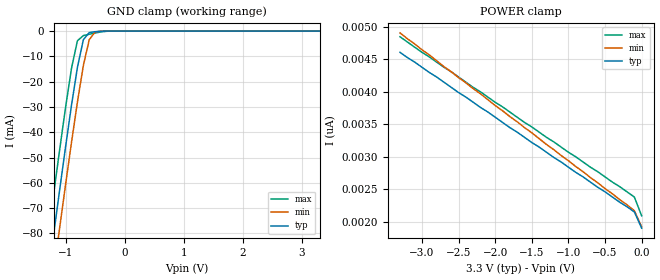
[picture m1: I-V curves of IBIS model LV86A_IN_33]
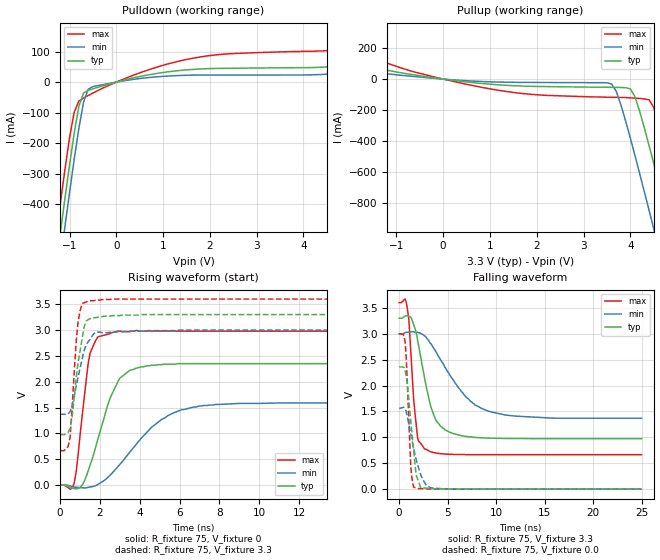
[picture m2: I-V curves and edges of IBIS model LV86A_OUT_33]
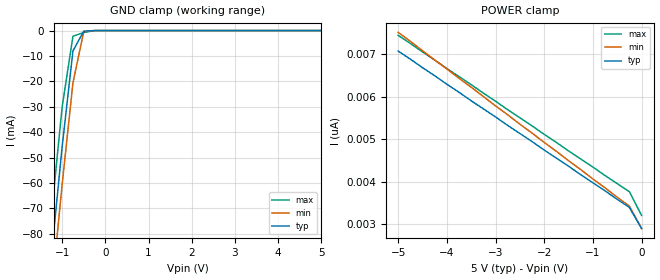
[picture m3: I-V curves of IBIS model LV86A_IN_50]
| TEXAS INSTRUMENTS INCORPORATED
| Standard Linear and Logic Group
| IBIS Model of SN74LV86A
| QUADRUPLE 2-INPUT EXCLUSIVE-OR GATE
| SOIC 14-pin (D), SOP 14-pin (NS), SSOP 14-pin (DB), TSSOP 14-pin (PW)
| and TVSOP 14-pin (DGV) Package
[IBIS Ver]   3.2
[Comment Char]  |_char
[File Name]   lv86a.ibs
[File Rev]   2.0 H_die
[Date]   May 24, 2000
[Source]   Data created from HSPICE simulations at TI-SLL.
[Notes]   The following is an IBIS list for the LV86A.
|   Please contact sllibis@ti.com with questions and
|   comments concerning SLL IBIS models.
[Disclaimer] Property of Texas Instruments Incorporated.  Unauthorized
   reproduction and/or distribution is strictly prohibited.
   This product is protected under copyright law.
   Created 2000, (C) Copyright 2000, Texas Instruments Inc.,
   All Rights Reserved.
   UNLESS THERE IS A SIGNED, WRITTEN AGREEMENT TO THE
   CONTRARY, TEXAS INSTRUMENTS () IS PROVIDING THE IBIS
   MODELS  AND WITHOUT ANY WARRANTY, EXPRESSED OR
   IMPLIED.  TI assumes no liability for:
   1) the accuracy of the IBIS models provided to your
   company;
   2) the proper functioning of these IBIS Models in your
   design or for any resulting applications; or
   3) infringement of patents, copyrights or intellectual
   property rights resulting from your use of these IBIS
   models.
   TI provides IBIS Models as a service to our customers.
   You and your company shall not distribute, sell or give
   these models to anyone else without prior written
   permission from TI.
   TI reserves the right to make changes to our products or
   to discontinue any semiconductor product or service
   without notice, and advises our customers to obtain the
   latest version of relevant information to verify, before
   placing orders, that the information being relied on is
   current.
   Please be aware that your receipt and use of the IBIS
   information provided shall serve as acceptance of these
   terms and conditions.  If you do not accept these terms,
   you should return or destroy the IBIS models and any
   other accompanying information immediately.
|   Component LV86A_D
[Component]   LV86A_D
[Manufacturer]  Texas Instruments, Inc.
[Package]
|   typ   min   max
R_pkg   0.031   0.028   0.034
L_pkg   3.109nH   2.462nH   3.889nH
C_pkg   0.473pF   0.363pF   0.628pF
[Pin]   signal_name   model_name   R_pin   L_pin   C_pin
1   1A   LV86A_IN   0.033   3.854nH   0.622pF
2   1B   LV86A_IN   0.032   3.188nH   0.473pF
3   1Y   LV86A_OUT   0.028   2.462nH   0.377pF
4   2A   LV86A_IN   0.031   2.596nH   0.363pF
5   2B   LV86A_IN   0.028   2.521nH   0.372pF
6   2Y   LV86A_OUT   0.034   3.250nH   0.476pF
7   GND   GND   0.034   3.889nH   0.628pF
8   3Y   LV86A_OUT   0.034   3.889nH   0.628pF
9   3A   LV86A_IN   0.034   3.250nH   0.476pF
10   3B   LV86A_IN   0.028   2.521nH   0.372pF
11   4Y   LV86A_OUT   0.031   2.596nH   0.364pF
12   4A   LV86A_IN   0.028   2.462nH   0.377pF
13   4B   LV86A_IN   0.032   3.188nH   0.473pF
14   VCC   POWER   0.033   3.854nH   0.622pF
|   Component LV86A_NS
[Component]   LV86A_NS
[Manufacturer]  Texas Instruments, Inc.
[Package]
|   typ   min   max
R_pkg   0.045   0.039   0.054
L_pkg   3.796nH   2.561nH   4.952nH
C_pkg   0.528pF   0.288pF   0.710pF
[Pin]   signal_name   model_name   R_pin   L_pin   C_pin
1   1A   LV86A_IN   0.047   4.867nH   0.706pF
2   1B   LV86A_IN   0.051   4.083nH   0.592pF
3   1Y   LV86A_OUT   0.041   2.915nH   0.376pF
4   2A   LV86A_IN   0.039   2.561nH   0.288pF
5   2B   LV86A_IN   0.041   3.101nH   0.430pF
6   2Y   LV86A_OUT   0.047   4.047nH   0.589pF
7   GND   GND   0.051   4.909nH   0.700pF
8   3Y   LV86A_OUT   0.045   4.784nH   0.694pF
9   3A   LV86A_IN   0.054   4.176nH   0.597pF
10   3B   LV86A_IN   0.039   3.287nH   0.449pF
11   4Y   LV86A_OUT   0.039   2.586nH   0.294pF
12   4A   LV86A_IN   0.040   2.802nH   0.371pF
13   4B   LV86A_IN   0.049   4.080nH   0.593pF
14   VCC   POWER   0.052   4.952nH   0.710pF
|   Component LV86A_DB
[Component]   LV86A_DB
[Manufacturer]  Texas Instruments, Inc.
[Package]
|   typ   min   max
R_pkg   0.044   0.041   0.046
L_pkg   3.551nH   3.258nH   3.927nH
C_pkg   0.402pF   0.360pF   0.421pF
[Pin]   signal_name   model_name   R_pin   L_pin   C_pin
1   1A   LV86A_IN   0.046   3.927nH   0.408pF
2   1B   LV86A_IN   0.044   3.587nH   0.421pF
3   1Y   LV86A_OUT   0.041   3.289nH   0.398pF
4   2A   LV86A_IN   0.042   3.258nH   0.360pF
5   2B   LV86A_IN   0.041   3.286nH   0.403pF
6   2Y   LV86A_OUT   0.044   3.586nH   0.421pF
7   GND   GND   0.046   3.927nH   0.408pF
8   3Y   LV86A_OUT   0.046   3.927nH   0.408pF
9   3A   LV86A_IN   0.044   3.586nH   0.421pF
10   3B   LV86A_IN   0.041   3.286nH   0.403pF
11   4Y   LV86A_OUT   0.043   3.258nH   0.360pF
12   4A   LV86A_IN   0.041   3.289nH   0.398pF
13   4B   LV86A_IN   0.044   3.587nH   0.421pF
14   VCC   POWER   0.046   3.927nH   0.408pF
|   Component LV86A_PW
[Component]   LV86A_PW
[Manufacturer]  Texas Instruments, Inc.
[Package]
|   typ   min   max
R_pkg   0.032   0.029   0.035
L_pkg   2.378nH   2.170nH   2.680nH
C_pkg   0.314pF   0.270pF   0.335pF
[Pin]   signal_name   model_name   R_pin   L_pin   C_pin
1   1A   LV86A_IN   0.033   2.618nH   0.330pF
2   1B   LV86A_IN   0.031   2.313nH   0.317pF
3   1Y   LV86A_OUT   0.030   2.310nH   0.314pF
4   2A   LV86A_IN   0.031   2.173nH   0.272pF
5   2B   LV86A_IN   0.030   2.204nH   0.309pF
6   2Y   LV86A_OUT   0.032   2.315nH   0.317pF
7   GND   GND   0.035   2.680nH   0.335pF
8   3Y   LV86A_OUT   0.033   2.640nH   0.333pF
9   3A   LV86A_IN   0.034   2.347nH   0.319pF
10   3B   LV86A_IN   0.029   2.277nH   0.313pF
11   4Y   LV86A_OUT   0.031   2.170nH   0.270pF
12   4A   LV86A_IN   0.031   2.244nH   0.311pF
13   4B   LV86A_IN   0.033   2.343nH   0.321pF
14   VCC   POWER   0.035   2.657nH   0.332pF
|   Component LV86A_DGV
[Component]   LV86A_DGV
[Manufacturer]  Texas Instruments, Inc.
[Package]
|   typ   min   max
R_pkg   0.035   0.020   0.045
L_pkg   2.499nH   2.077nH   2.966nH
C_pkg   0.361pF   0.305pF   0.416pF
[Pin]   signal_name   model_name   R_pin   L_pin   C_pin
1   1A   LV86A_IN   0.027   2.717nH   0.373pF
2   1B   LV86A_IN   0.037   2.434nH   0.398pF
3   1Y   LV86A_OUT   0.034   2.200nH   0.316pF
4   2A   LV86A_IN   0.020   2.077nH   0.309pF
5   2B   LV86A_IN   0.030   2.147nH   0.305pF
6   2Y   LV86A_OUT   0.042   2.580nH   0.408pF
7   GND   GND   0.039   2.921nH   0.385pF
8   3Y   LV86A_OUT   0.033   2.841nH   0.380pF
9   3A   LV86A_IN   0.042   2.611nH   0.410pF
10   3B   LV86A_IN   0.038   2.331nH   0.329pF
11   4Y   LV86A_OUT   0.026   2.223nH   0.319pF
12   4A   LV86A_IN   0.034   2.259nH   0.313pF
13   4B   LV86A_IN   0.045   2.681nH   0.416pF
14   VCC   POWER   0.042   2.966nH   0.386pF
[Model Selector]   LV86A_IN
LV86A_IN_33   3.3-V Vcc Input Model
LV86A_IN_50   5.0-V Vcc Input Model
[Model Selector]   LV86A_OUT
LV86A_OUT_33   3.3-V Vcc Output Model
LV86A_OUT_50   5.0-V Vcc Output Model
| Models and submodels in the file (4): LV86A_IN_33 (Input), LV86A_OUT_33 (Output), LV86A_IN_50 (Input), LV86A_OUT_50 (Output)
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|   Model LV86A_IN_33
[Model]   LV86A_IN_33
Model_type  Input
Polarity   Inverting
Vinl = 0.99
Vinh = 2.31
| variable   typ   min   max
C_comp   1.24pf   0.94pf   1.54pf
[Temperature Range]   25   85   -40
[Voltage Range]   3.3   3.0   3.6
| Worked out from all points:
|   GND clamp passes 1 mA (typ) near -0.61 V on its own axis
[GND Clamp]
|   Voltage   I(typ)   I(min)   I(max)
-3.3V     -460mA     -475mA     -445mA
-1.3V     -97.5mA    -113mA     -81.5mA
-1.2V     -79.9mA    -95mA      -63.9mA
-1.1V     -62.6mA    -77.6mA    -46.7mA
-1V       -45.6mA    -60.5mA    -30mA
-900mV    -29.2mA    -43.9mA    -14.6mA
-800mV    -14.3mA    -28mA      -3.81mA
-700mV    -3.42mA    -13.6mA    -1.78mA
-600mV    -581uA     -3.4mA     -1.25mA
-500mV    -233uA     -353uA     -759uA
-400mV    -58.1uA    -21.9uA    -324uA
3.3V      1.9nA      2.34nA     1.69nA
[POWER Clamp]
|   Voltage   I(typ)   I(min)   I(max)
-3.3V     4.61nA     4.91nA     4.85nA
-3V       4.38nA     4.65nA     4.61nA
-100mV    2.15nA     2.17nA     2.38nA
0V        1.9nA      1.92nA     2.09nA
|   Model LV86A_OUT_33
[Model]   LV86A_OUT_33
Model_type  Output
Polarity   Non-Inverting
Vmeas = 1.65v
Cref = 15pf
| variable   typ   min   max
C_comp   4.62pf   3.47pf   5.77pf
[Temperature Range]   25   85   -40
[Voltage Range]   3.3   3.0   3.6
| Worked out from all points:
|   slope of the pulldown table from 0 to 0.495 V, typ, clamps not added: 27.3 ohm
|   slope of the pullup table from 0 to 0.495 V, typ, clamps not added: 27.2 ohm
|   rising waveform, R_fixture 75, V_fixture 0: 20-80 % time 1.17ns typ, 2.3ns min, 519ps max; typ from 0 V to 2.35 V
|   falling waveform, R_fixture 75, V_fixture 3.3: 20-80 % time 1.61ns typ, 3.65ns min, 668ps max; typ from 3.3 V to 0.976 V
|   rising waveform, R_fixture 75, V_fixture 3.3: 20-80 % time 471ps typ, 570ps min, 307ps max; typ from 0.976 V to 3.3 V
|   falling waveform, R_fixture 75, V_fixture 0.0: 20-80 % time 721ps typ, 1.16ns min, 400ps max; typ from 2.36 V to 0 V
[Pulldown]
|   Voltage   I(typ)   I(min)   I(max)
-3.3V     -3.04A     -3.13A     -2.95A
-1.3V     -615mA     -707mA     -518mA
-1.2V     -498mA     -591mA     -401mA
-1.1V     -383mA     -475mA     -288mA
-900mV    -167mA     -253mA     -98.6mA
-800mV    -79.1mA    -151mA     -61.7mA
-700mV    -35.5mA    -66.4mA    -51.9mA
-600mV    -26.8mA    -23.2mA    -43.9mA
-500mV    -22mA      -14.7mA    -35.8mA
1.6V      41.2mA     22.8mA     77.1mA
4.7V      52.3mA     27.8mA     106mA
6.6V      95.5mA     55.2mA     176mA
[Pullup]
|   Voltage   I(typ)   I(min)   I(max)
-3.3V     177mA      99.8mA     326mA
500mV     -18.4mA    -10.6mA    -33.4mA
3.6V      -52.9mA    -31.5mA    -117mA
3.8V      -54.2mA    -168mA     -119mA
4V        -62.6mA    -381mA     -121mA
4.1V      -115mA     -494mA     -123mA
4.4V      -429mA     -845mA     -133mA
4.5V      -544mA     -964mA     -182mA
4.8V      -899mA     -1.32A     -505mA
4.9V      -1.02A     -1.44A     -622mA
5.2V      -1.38A     -1.81A     -981mA
6.6V      -3.09A     -3.52A     -2.69A
[Ramp]
| variable   typ   min   max
dV/dt_r   1.42E+00/1.13E-09   9.68E-01/2.37E-09   1.80E+00/5.02E-10
dV/dt_f   1.43E+00/1.59E-09   1.00E+00/3.74E-09   1.80E+00/6.48E-10
R_load = 75
[Rising Waveform]
R_fixture = 75
V_fixture = 0
|   Time   V(typ)   V(min)   V(max)
0s        0V         0V         0V
700ps     -67.3mV    -36.6mV    31.2mV
1.4ns     268mV      -45.9mV    2.33V
1.9ns     897mV      14.4mV     2.87V
2.5ns     1.67V      188mV      2.93V
3ns       2.07V      400mV      2.98V
4.4ns     2.31V      1.04V      2.98V
5.7ns     2.34V      1.4V       2.98V
7.8ns     2.35V      1.56V      2.98V
25ns      2.35V      1.59V      2.98V
[Falling Waveform]
R_fixture = 75
V_fixture = 3.3
V_fixture_min = 3.0
V_fixture_max = 3.6
|   Time   V(typ)   V(min)   V(max)
0s        3.3V       3V         3.6V
800ps     3.35V      3.03V      3.54V
1ns       3.34V      3.03V      3.28V
1.5ns     3.17V      3.04V      1.72V
1.9ns     2.88V      3.03V      994mV
2.6ns     2.17V      2.96V      782mV
3.3ns     1.57V      2.8V       719mV
4.3ns     1.21V      2.49V      685mV
9ns       987mV      1.52V      666mV
25ns      976mV      1.37V      666mV
[Rising Waveform]
R_fixture = 75
V_fixture = 3.3
V_fixture_min = 3.0
V_fixture_max = 3.6
|   Time   V(typ)   V(min)   V(max)
0s        976mV      1.37V      666mV
400ps     1.02V      1.38V      746mV
500ps     1.09V      1.42V      919mV
800ps     2.05V      1.9V       2.75V
900ps     2.37V      2.09V      3.16V
1.1ns     2.82V      2.43V      3.51V
1.4ns     3.2V       2.77V      3.56V
1.8ns     3.24V      2.96V      3.58V
4.4ns     3.3V       2.99V      3.6V
25ns      3.3V       3V         3.6V
[Falling Waveform]
R_fixture = 75
V_fixture = 0.0
|   Time   V(typ)   V(min)   V(max)
0s        2.36V      1.56V      3V
600ps     2.3V       1.56V      2.86V
700ps     2.21V      1.51V      2.65V
800ps     2.1V       1.44V      2.25V
1.2ns     1.3V       1.06V      439mV
1.5ns     734mV      787mV      38.7mV
1.8ns     245mV      537mV      20.4mV
2.2ns     43.3mV     291mV      10.9mV
3.3ns     9.4mV      24.5mV     3.33mV
25ns      0V         1.05uV     4.84uV
|   Model LV86A_IN_50
[Model]   LV86A_IN_50
Model_type  Input
Polarity   Inverting
Vinl = 1.5
Vinh = 3.5
| variable   typ   min   max
C_comp   1.24pf   0.94pf   1.54pf
[Temperature Range]   25   85   -40
[Voltage Range]   5.0   4.5   5.5
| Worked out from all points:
|   GND clamp passes 1 mA (typ) near -0.52 V on its own axis
[GND Clamp]
|   Voltage   I(typ)   I(min)   I(max)
-5V       -773mA     -786mA     -758mA
-1.5V     -133mA     -148mA     -117mA
-1.25V    -88.7mA    -104mA     -72.7mA
-1V       -45.6mA    -60.5mA    -30mA
-750mV    -7.99mA    -20.5mA    -2.23mA
-500mV    -233uA     -353uA     -759uA
-250mV    -2.63nA    -182nA     -26.9uA
5V        2.9nA      3.64nA     2.54nA
[POWER Clamp]
|   Voltage   I(typ)   I(min)   I(max)
-5V       7.08nA     7.52nA     7.45nA
-1.5V     4.37nA     4.5nA      4.73nA
-250mV    3.4nA      3.43nA     3.77nA
0V        2.9nA      2.91nA     3.21nA
